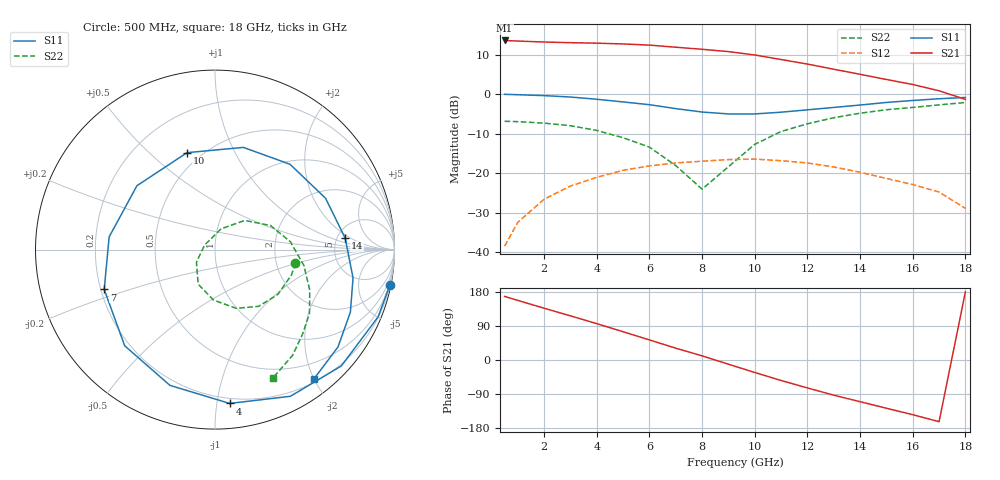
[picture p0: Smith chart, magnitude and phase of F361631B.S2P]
!ATF-36163
!1.5V 15mA
! last updated 11-10-95
# ghz s ma r 50
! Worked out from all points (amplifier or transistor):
!   19 points, 500 MHz to 18 GHz, reference 50 ohm
!   highest |S21| = 13.6 dB at 500 MHz (marker M1)
!   |S21| within 3 dB of that: start of sweep to 9.213 GHz
!   unconditionally stable (mu >= 1): 10.65 GHz to end of sweep
!   at 3 GHz: K = 0.35, MSG = 18.1 dB, |S12| = -23.2 dB
!   at 9 GHz: K = 0.90, MSG = 13.6 dB, |S12| = -16.5 dB
!   at 18 GHz: K = 1.69, MAG = 8.9 dB, |S12| = -28.9 dB
!   lowest NFmin = 0.49 dB at 2 GHz
!   S11 on the Smith chart (normalised r, x): 500 MHz: 0.29, -9.84; 4 GHz: 0.16, -1.09; 7 GHz: 0.21, -0.17; 10 GHz: 0.42, +0.66; 14 GHz: 5.90, +1.61; 18 GHz: 0.25, -2.00
0.5  0.994 -11.6  4.763 167.8  0.012 79.4  0.454 -9.4
1  0.983 -22.4  4.68 157.2  0.024 71.3  0.449 -18.3
2  0.957 -42.6  4.55 136.7  0.047 55.8  0.43 -35.5
3  0.919 -62.8  4.465 116.5  0.069 40.4  0.399 -52.4
4  0.861 -84.5  4.402 95.9  0.089 23.9  0.348 -70.1
5  0.797 -108.4  4.303 74.6  0.109 6.5  0.281 -91.8
6  0.735 -133.2  4.16 53.0  0.124 -10.6  0.214 -116.0
7  0.656 -160.2  3.911 31.2  0.135 -28.4  0.125 -145.8
8  0.594 173.2  3.684 10.9  0.142 -42.2  0.063 155.8
9  0.562 140.7  3.443 -11.1  0.149 -57.6  0.121 73.4
10  0.562 106.1  3.122 -32.9  0.151 -73.5  0.232 44.4
11  0.591 74.5  2.736 -54.0  0.144 -88.4  0.337 23.5
12  0.633 48.7  2.397 -73.7  0.135 -101.6  0.422 6.0
13  0.679 25.0  2.063 -92.8  0.12 -114.6  0.503 -10.1
14  0.728 5.1  1.78 -110.0  0.103 -124.0  0.574 -23.1
15  0.785 -11.6  1.531 -127.3  0.086 -133.3  0.635 -34.0
16  0.831 -24.8  1.323 -144.3  0.072 -139.3  0.679 -44.1
17  0.874 -38.4  1.102 -162.8  0.058 -147.7  0.731 -53.8
18  0.907 -52.5  0.858 179.7  0.036 -154.9  0.784 -65.6
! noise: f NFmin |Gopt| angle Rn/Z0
2  0.49  0.84  28.13  0.376
3  0.54  0.744  42  0.313
5  0.63  0.586  72.09  0.193
7  0.73  0.464  105.6  0.112
9  0.85  0.304  140  0.075
10  0.91  0.206  174.2  0.075
12  1.07  0.199  -82.86  0.138
14  1.27  0.375  -12.44  0.338
16  1.54  0.595  21.02  0.642
18  1.93  0.712  52.09  1.184
